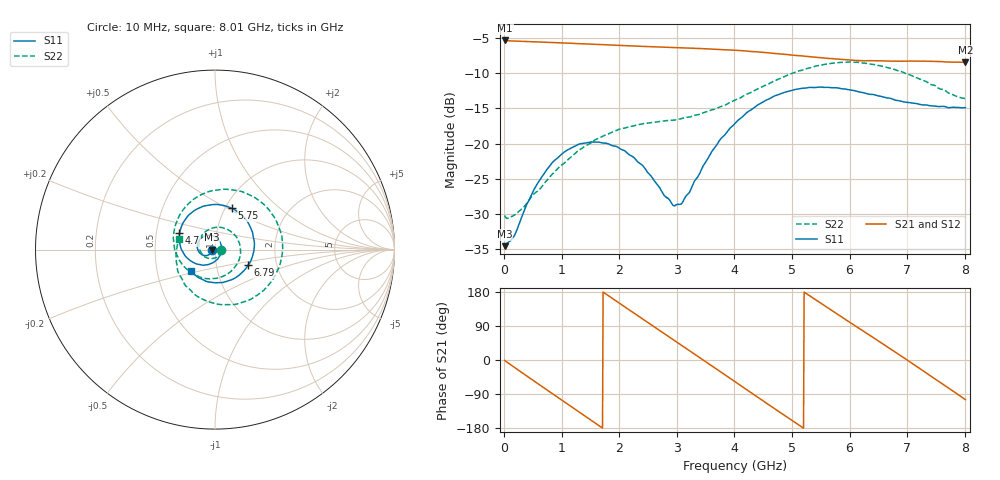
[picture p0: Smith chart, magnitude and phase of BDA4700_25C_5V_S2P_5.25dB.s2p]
!Agilent Technologies,E5071B,MY42404982,A.09.10
!Date: Mon Oct 20 13:28:32 2025
!Data & Calibration Information:
!Freq	S11:SOLT2(ON)	S21:SOLT2(ON)	S12:SOLT2(ON)	S22:SOLT2(ON)
# Hz S RI R 50
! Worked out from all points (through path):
!   801 points, 10 MHz to 8.01 GHz, reference 50 ohm
!   highest |S21| = -5.37 dB at 20 MHz (marker M1); lowest = -8.5 dB at 8.01 GHz (marker M2)
!   group delay of S21, straight-line fit = 285 ps
!   lowest |S11| = -34.5 dB at 10 MHz (marker M3), VSWR 1.04, Z = 48.2 - j0.105 ohm
!   |S11| at or under -10 dB: start of sweep to end of sweep
!   |S22| runs from -30.6 to -8.4 dB; largest |S21 - S12| = 0.0043
!   S11 on the Smith chart (normalised r, x): 10 MHz: 0.96, -0.00; 4.7 GHz: 0.66, +0.13; 5.75 GHz: 1.08, +0.53; 6.79 GHz: 1.42, -0.26; 8.01 GHz: 0.74, -0.18
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1e7  -0.0187 -0.00109  0.5385 -0.0115  0.5388 -0.012  0.0309 -0.00259
2e7  -0.0192 -0.00195  0.5383 -0.0211  0.5384 -0.0227  0.0303 -0.00271
3.4e8  -0.0252 -0.0208  0.4269 -0.3147  0.4269 -0.3153  0.0211 -0.0286
7.2e8  -0.0537 -0.0336  0.1227 -0.5084  0.123 -0.5087  -0.0177 -0.0505
1.02e9  -0.083 -0.0208  -0.1582 -0.4925  -0.1584 -0.4926  -0.0621 -0.0355
1.35e9  -0.0992 0.0144  -0.4038 -0.3125  -0.4042 -0.3126  -0.0896 0.023
1.93e9  -0.0592 0.0755  -0.4604 0.1912  -0.4605 0.1913  -0.00206 0.1228
2.32e9  -0.00752 0.074  -0.2243 0.4365  -0.2243 0.4367  0.1008 0.0911
2.68e9  0.0289 0.0411  0.0832 0.4779  0.0831 0.4776  0.1429 -0.00946
3.04e9  0.0352 -0.0117  0.35 0.3261  0.3491 0.3272  0.0982 -0.1124
3.37e9  0.00768 -0.0583  0.467 0.0739  0.4672 0.0735  0.00273 -0.1604
4.01e9  -0.1183 -0.0732  0.2484 -0.386  0.2484 -0.3858  -0.1906 -0.0713
4.35e9  -0.1812 -0.0104  -0.0191 -0.448  -0.0194 -0.4488  -0.2314 0.0562
4.7e9  -0.1979 0.092  -0.2727 -0.3401  -0.2721 -0.3407  -0.1898 0.2044
5.35e9  -0.051 0.2449  -0.3974 0.1074  -0.398 0.1064  0.1052 0.3311
5.75e9  0.0958 0.23  -0.2272 0.3276  -0.2266 0.3279  0.3019 0.22
6.19e9  0.2025 0.113  0.0598 0.3829  0.063 0.3833  0.3734 -0.0295
6.68e9  0.2027 -0.0556  0.326 0.2044  0.3269 0.2038  0.223 -0.262
6.79e9  0.1838 -0.0871  0.3586 0.1381  0.3596 0.1364  0.1688 -0.2885
7.3e9  0.0532 -0.1807  0.3293 -0.1978  0.3291 -0.1986  -0.0985 -0.2608
7.66e9  -0.0523 -0.1749  0.1407 -0.3525  0.1402 -0.3532  -0.208 -0.1144
8.01e9  -0.1351 -0.1191  -0.0953 -0.3641  -0.0951 -0.3646  -0.2009 0.057
